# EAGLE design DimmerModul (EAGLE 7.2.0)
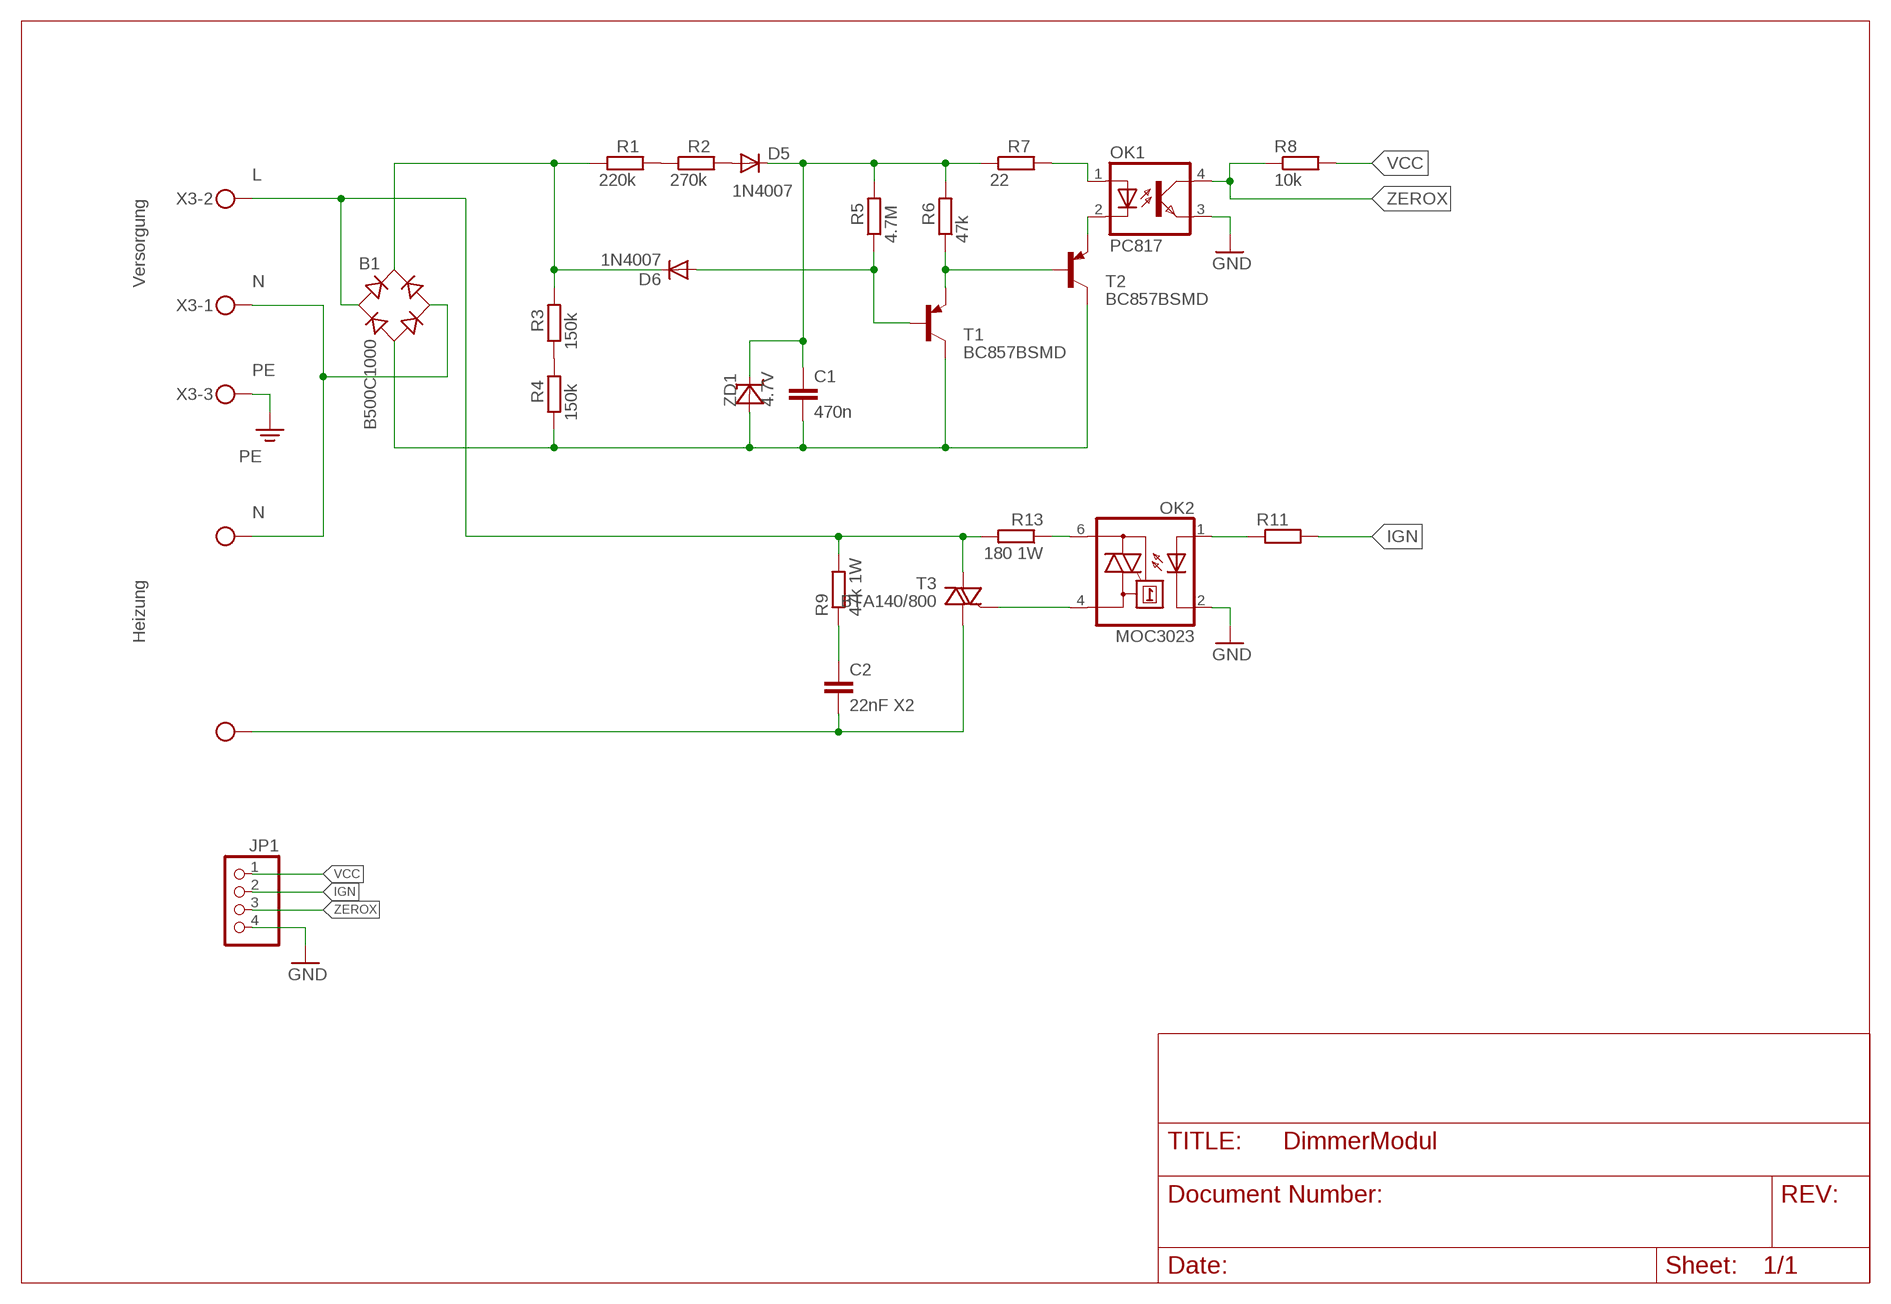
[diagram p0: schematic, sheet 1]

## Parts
B1  B500C1000  B-DIL  [B-DIL]
C1  470n  C_1206  [1206]
C2  22nF X2  C-EU150-054X183  [C150-054X183]
D5  1N4007  DIODE-MELF-MLL41  [MELF-MLL41]
D6  1N4007  DIODE-MELF-MLL41  [MELF-MLL41]
JP1  PINHD-1X4  [1X04]
OK1  PC817  [DIL04]
OK2  MOC3023  MOC3023M  [DIL06]
R1  220k  R_1206  [1206]
R2  270k  R_1206  [1206]
R3  150k  R_1206  [1206]
R4  150k  R_1206  [1206]
R5  4.7M  R_1206  [1206]
R6  47k  R_1206  [1206]
R7  22  R_1206  [1206]
R8  10k  R_0805  [0805]
R9  47k 1W  R-EU_0207/10  [0207/10]
R11  R_0805  [0805]
R13  180 1W  R-EU_0207/7  [0207/7]
T1  BC857BSMD  [SOT23-BEC]
T2  BC857BSMD  [SOT23-BEC]
T3  BTA140/800  TIC225S  [TO220DS]
X2  MKDSN1,5/2-5,08  [MKDSN1,5/2-5,08]
X3  MKDSN1,5/3-5,08  [MKDSN1,5/3-5,08]
ZD1  4.7V  ZF4,3  [MINIMELF]

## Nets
GND: JP1.4 OK1.3(EMIT) OK2.2(C)
IGN: JP1.2 R11.P$2
L: B1.AC1 R9.2 R13.2 T3.A2 X3.2
N: B1.AC2 X2.1 X3.1
N$1: R1.P$2 R2.P$1
N$2: D5.A R2.P$2
N$3: R3.P$1 R4.P$2
N$4: B1.+ D6.C R1.P$1 R3.P$2
N$5: OK2.1(A) R11.P$1
N$6: OK2.6(A2) R13.1
N$7: B1.- C1.P$2 R4.P$1 T1.C T2.C ZD1.A
N$8: D6.A R5.P$1 T1.B
N$9: C1.P$1 D5.C R5.P$2 R6.P$2 R7.P$1 ZD1.C
N$10: R6.P$1 T1.E T2.B
N$11: OK1.1(A) R7.P$2
N$12: OK1.2(C) T2.E
N$13: OK2.4(A1) T3.G
N$20: C2.1 R9.1
N$21: C2.2 T3.A1 X2.2
PE: X3.3
VCC: JP1.1 R8.P$2
ZEROX: JP1.3 OK1.4(COL) R8.P$1

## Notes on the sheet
- Versorgung
- Heizung

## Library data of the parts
B1 = rectifier:B-DIL: RECTIFIER
C1 = smd_rcl:C
C2 = rcl:C-EU: CAPACITOR, European symbol
D5 D6 = diode:DIODE-: DIODE
JP1 = pinhead:PINHD-1X4: PIN HEADER
OK1 = optocoupler:PC817: SHARP OPTO COUPLER; MPN: PC817X4J000F; OC_FARNELL: 9707727; OC_NEWARK: 97K7059
OK2 = optocoupler:MOC30*M: RANDOM-PHASE OPTOISOLATORS TRIAC DRIVER OUTPUT Source: http://www.fairchildsemi.com MOC3020-M.pdf; MF: FAIRCHILD SEMICONDUCTOR; MPN: MOC3023-M; OC_FARNELL: 1021367; OC_NEWARK: 72K8896
R1-R8 R11 = smd_rcl:R
R9 R13 = rcl:R-EU_: RESISTOR, European symbol
T1 T2 = transistor-pnp:BC857*: PNP Transistror
T3 = triac:TIC225S: TRIAC
X2 = con-phoenix-508:MKDSN1,5/2-5,08: MKDSN 1,5/ 2-5,08 Printklemme
X3 = con-phoenix-508:MKDSN1,5/3-5,08: MKDSN 1,5/ 3-5,08 Printklemme Nennstrom: 13,5 A Nennspannung: 250 V Rastermaß: 5,08 mm Polzahl: 3 Anschlussart: Schraubanschluss Montage: Löten Anschlussrichtung Leiter/Platine: 0 ° Artikelnummer: 1729131 Source: http://eshop.phoenixcontact.com .. 1729131.pdf
ZD1 = smd_diode:ZF4,3

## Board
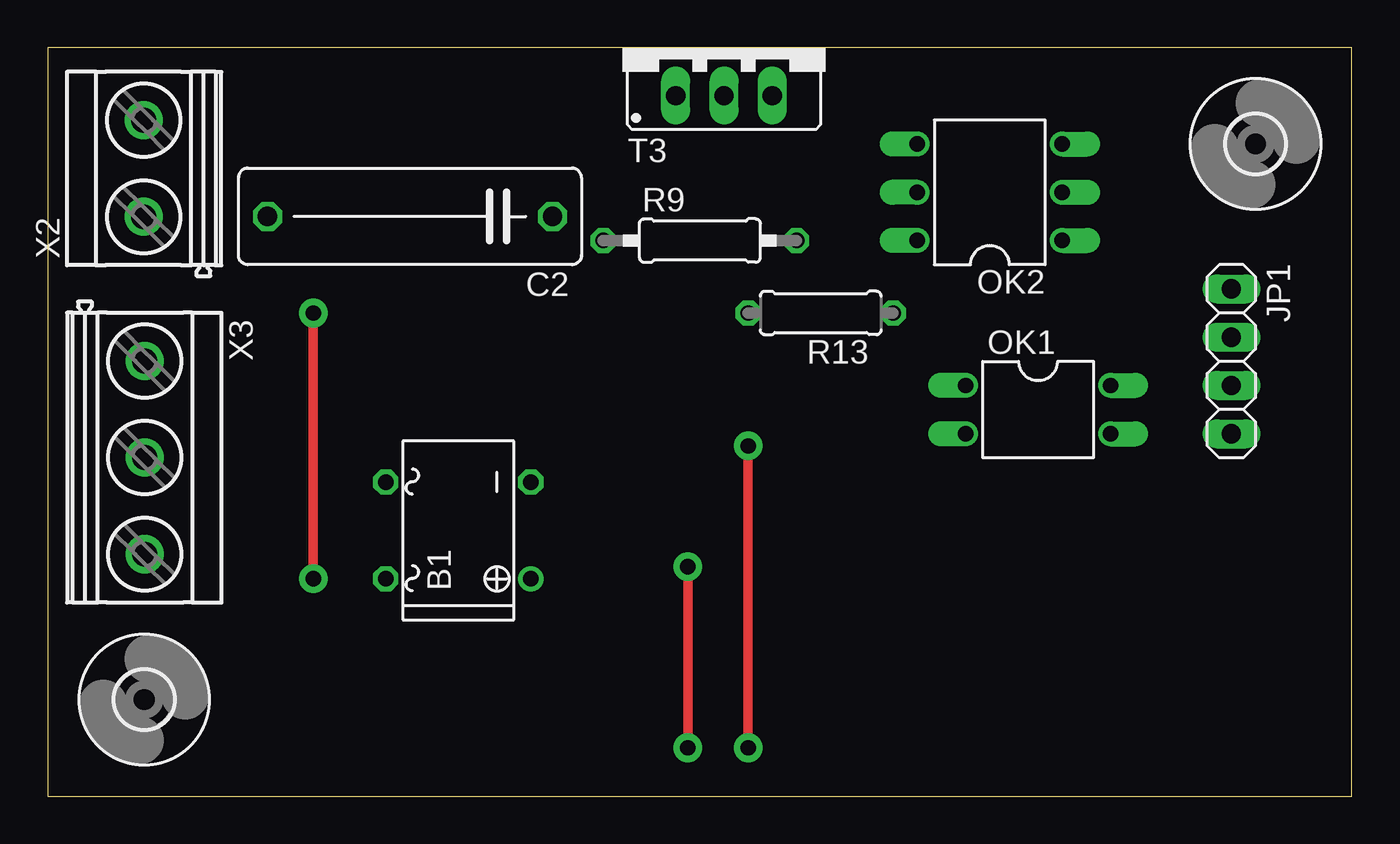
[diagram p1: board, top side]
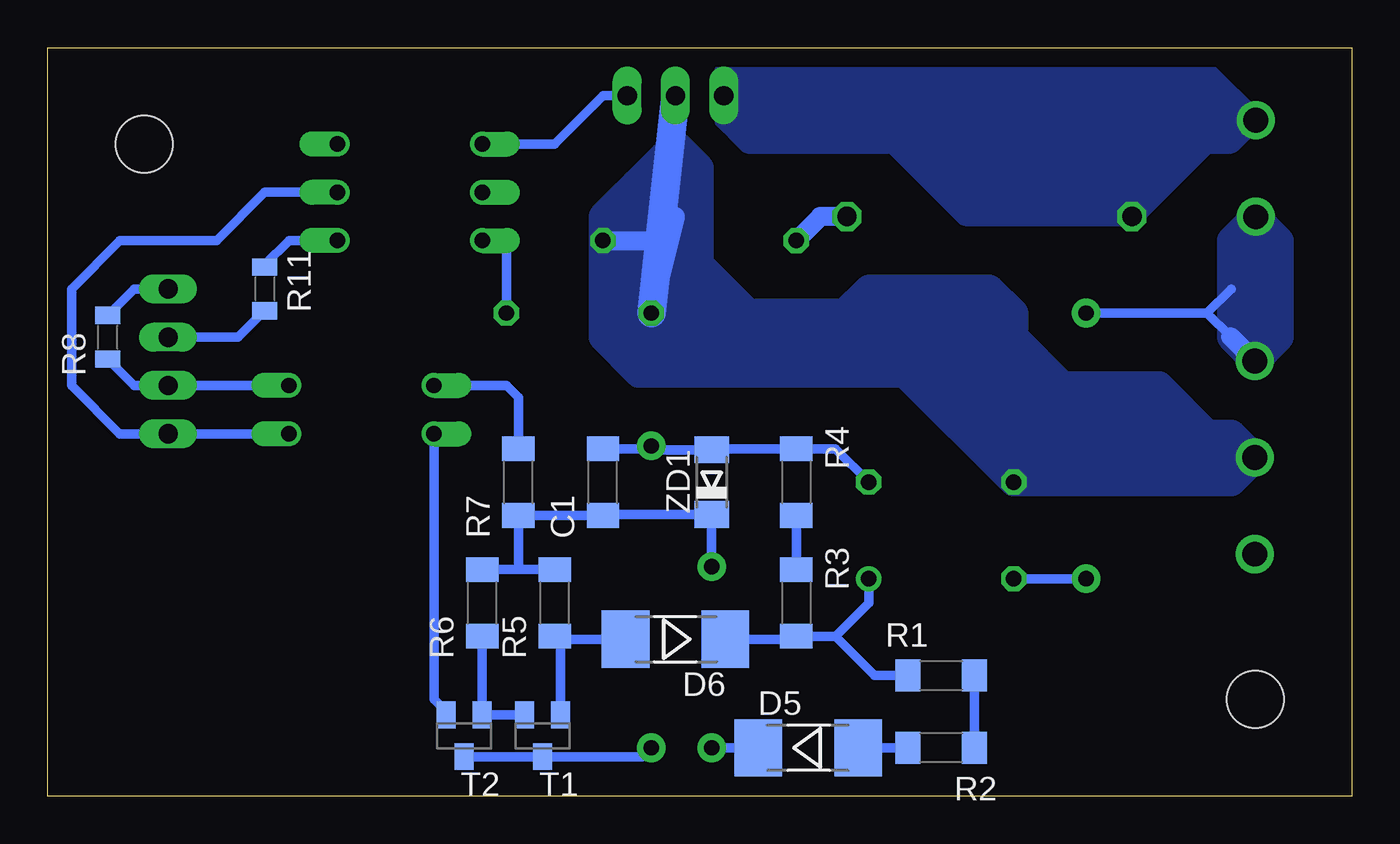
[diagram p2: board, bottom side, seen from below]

Size 68.57 x 39.36 mm. Coordinates in mm from the lower left corner, seen from the top.
Outline: 0,0 68.57,0 68.57,39.36 0,39.36 0,0
Copper layers (1*16): Top 0.035mm / dielectric 1.5mm / Bottom 0.035mm
Design rules "default": minimum track width 10mil, minimum drill 24mil, track to track 8mil, track to pad 8mil, pad to pad 8mil, via to via 8mil, smd to smd 8mil, copper to edge 40mil, drill to drill 8mil, minimum pad ring 10mil, minimum via ring 8mil, stop-mask expansion 4mil, vias tented up to drill 0mil, thermal gap 10mil

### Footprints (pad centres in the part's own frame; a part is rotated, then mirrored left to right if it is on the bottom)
B-DIL = drill 0.813: + -2.54,-3.81 | drill 0.813 octagon: - 2.54,-3.81; AC1 2.54,3.81; AC2 -2.54,3.81
1206 = smd 1.3 x 1.7: P$1 -1.75,0; P$2 1.75,0
C150-054X183 = drill 1.016 octagon: 1 -7.493,0; 2 7.493,0
MELF-MLL41 = smd 2.5 x 3: A 2.625,0; C -2.625,0
1X04 = drill 1.016 long: 1 -3.81,0; 2 -1.27,0; 3 1.27,0; 4 3.81,0
DIL04 = drill 0.813 offset: 1 -1.27,-3.81; 2 1.27,-3.81; 3 1.27,3.81; 4 -1.27,3.81
DIL06 = drill 0.813 offset: 1 -2.54,-3.81; 2 0,-3.81; 3 2.54,-3.81; 4 2.54,3.81; 5 0,3.81; 6 -2.54,3.81
0805 = smd 0.9 x 1.3: P$1 -1.15,0; P$2 1.15,0
0207/10 = drill 0.813 octagon: 1 -5.08,0; 2 5.08,0
0207/7 = drill 0.813 octagon: 1 -3.81,0; 2 3.81,0
SOT23-BEC = smd 1 x 1.4: B -0.95,-1.1; C 0,1.1; E 0.95,-1.1
TO220DS = drill 1.016 long: A1 -2.54,-2.54; A2 0,-2.54; G 2.54,-2.54
3,0 = hole 3: 0,0
MKDSN1,5/2-5,08 = drill 1.3 pad 2: 1 -2.561,0.025; 2 2.519,0.025
MKDSN1,5/3-5,08 = drill 1.3 pad 2: 1 -7.641,0.025; 2 -2.561,0.025; 3 2.519,0.025
MINIMELF = smd 1.4 x 1.8: A 1.7,0; C -1.7,0

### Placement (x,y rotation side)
B1  21.59,13.97 90 top
C1  39.37,16.51 90 bottom
C2  19.05,30.48 180 top
D5  28.57,2.54 0 bottom
D6  35.56,8.26 180 bottom
JP1  62.23,22.86 270 top
OK1  52.07,20.32 270 top
OK2  49.53,31.75 90 top
R1  21.59,6.35 0 bottom
R2  21.59,2.54 180 bottom
R3  29.21,10.16 270 bottom
R4  29.21,16.51 270 bottom
R5  41.91,10.16 90 bottom
R6  45.72,10.16 90 bottom
R7  43.81,16.51 90 bottom
R8  65.41,24.13 90 bottom
R9  34.29,29.21 0 top
R11  57.15,26.67 270 bottom
R13  40.64,25.4 180 top
T1  42.55,3.18 180 bottom
T2  46.67,3.18 180 bottom
T3  35.56,39.37 0 top
U$1  [3,0]  5.08,5.08 0 top
U$2  [3,0]  63.5,34.29 0 top
X2  5.08,33.02 90 top
X3  5.08,15.24 270 top
ZD1  33.66,16.51 90 bottom

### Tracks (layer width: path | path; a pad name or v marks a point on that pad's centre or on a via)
GND
  Bottom 0.5: OK2.2 57.15,31.75 59.69,29.21 64.77,29.21 67.31,26.67 67.31,21.59 64.77,19.05 JP1.4 OK1.3
IGN
  Bottom 0.5: JP1.2 58.54,24.13 R11.P$2
L
  Bottom 1: R9.2 36.83,29.21 35.56,30.48 R13.2
  Bottom 1.5: T3.A2 R13.2
  pour Bottom (no thermals): 39.37,30.48 39.37,24.13 37.47,22.23 23.5,22.23 17.78,16.51 6.35,16.51 5.08,17.78 6.35,19.05 7.62,19.05 10.16,21.59 15.24,21.59 17.78,24.13 17.78,25.4 19.05,26.67 25.4,26.67 26.67,25.4 31.75,25.4 34.29,27.94 34.29,33.02 35.56,34.29
N  (via drill 0.8 pad 1.5)
  Top 0.5: v13.97,11.43 v13.97,25.4
  Bottom 0.5: 6.38,24.16 7.62,25.4 | v13.97,25.4 7.62,25.4 | 7.62,25.4 6.35,26.67 | v13.97,11.43 B1.AC2
  Bottom 1: X3.1 6.38,24.16
  pour Bottom (no thermals): 5.08,22.86 3.81,24.13 3.81,29.21 5.08,30.48 6.35,29.21 6.35,24.13
N$1
  Bottom 0.5: R1.P$2 R2.P$1
N$2
  Bottom 0.5: R2.P$2 D5.A
N$3
  Bottom 0.5: R3.P$1 R4.P$2
N$4
  Bottom 0.5: D6.C 29.36,8.26 R3.P$2 27.15,8.41 | 27.15,8.41 25.4,10.16 B1.+ | R1.P$1 25.09,6.35 27.15,8.41
N$5
  Bottom 0.5: OK2.1 55.88,29.21 57.15,27.94 R11.P$1
N$6
  Bottom 0.5: OK2.6 44.45,29.21 R13.1
N$7  (via drill 0.8 pad 1.5)
  Top 0.5: v36.83,18.41 v36.83,2.54
  Bottom 0.5: B1.- 27.15,18.26 R4.P$1 33.02,18.26 33.07,18.21 ZD1.A 36.62,18.21 v36.83,18.41 36.98,18.26 C1.P$2 | T2.C T1.C 37.3,2.08 v36.83,2.54
N$8
  Bottom 0.5: 37.78,7.86 D6.A 41.76,8.26 R5.P$1 41.59,8.1 T1.B
N$9  (via drill 0.8 pad 1.5)
  Top 0.5: v33.66,2.54 v33.66,12.07
  Bottom 0.5: D5.C v33.66,2.54 | v33.66,12.07 ZD1.C 39.32,14.81 C1.P$1 R7.P$1 43.81,11.91 | R5.P$2 43.81,11.91 | 43.81,11.91 R6.P$2
N$10
  Bottom 0.5: R6.P$1 T2.B T1.E
N$11
  Bottom 0.5: R7.P$2 43.81,20.96 44.45,21.59 OK1.1
N$12
  Bottom 0.5: T2.E 47.62,4.44 48.26,5.08 OK1.2
N$13
  Bottom 0.5: T3.G 39.37,36.83 41.91,34.29 OK2.4
N$20
  Bottom 1: C2.1 27.94,30.48 R9.1
N$21
  pour Bottom (no thermals): 11.43,30.48 7.62,34.29 6.35,34.29 5.08,35.56 7.62,38.1 33.02,38.1 33.02,35.56 31.75,34.29 24.13,34.29 20.32,30.48
VCC
  Bottom 0.5: JP1.1 64.02,26.67 R8.P$2
ZEROX
  Bottom 0.5: R8.P$1 64.02,21.59 JP1.3 OK1.4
